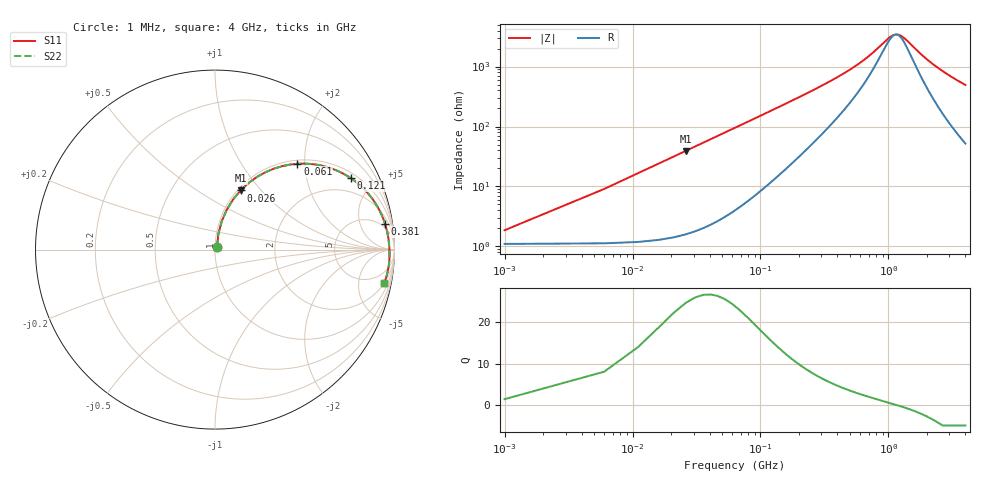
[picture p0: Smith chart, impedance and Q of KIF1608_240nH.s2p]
# MHz S RI R 50
!Freq ReS11 ImS11 ReS21 ImS21 ReS12 ImS12 ReS22 ImS22
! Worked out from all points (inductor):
!   801 points, 1 MHz to 4 GHz, reference 50 ohm
!   read as one part in series: L = 239 nH near 21 MHz
!   highest Q = 23.4 at 26 MHz (marker M1), where L = 239 nH
!   self-resonance near 1.146 GHz
!   S11 on the Smith chart (normalised r, x): 1 MHz: 1.02, +0.03; 26 MHz: 1.03, +0.78; 61 MHz: 1.08, +1.84; 121 MHz: 1.24, +3.66; 381 MHz: 4, +12; 4 GHz: 2, -10
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1  0.0111 0.0147  0.9889 -0.0147  0.9889 -0.0147  0.0111 0.0147
11  0.0374 0.1572  0.9626 -0.1572  0.9626 -0.1572  0.0374 0.1572
26  0.1424 0.3298  0.8576 -0.3298  0.8576 -0.3298  0.1424 0.3298
31  0.1877 0.3718  0.8123 -0.3718  0.8123 -0.3718  0.1877 0.3718
41  0.2829 0.4321  0.7171 -0.4321  0.7171 -0.4321  0.2829 0.4321
61  0.4594 0.4782  0.5406 -0.4782  0.5406 -0.4782  0.4594 0.4782
91  0.6467 0.4528  0.3533 -0.4528  0.3533 -0.4528  0.6467 0.4528
121  0.7572 0.3978  0.2428 -0.3978  0.2428 -0.3978  0.7572 0.3978
161  0.8386 0.3287  0.1614 -0.3287  0.1614 -0.3287  0.8386 0.3287
211  0.8907 0.2628  0.1093 -0.2628  0.1093 -0.2628  0.8907 0.2628
286  0.9273 0.1961  0.0727 -0.1961  0.0727 -0.1961  0.9273 0.1961
381  0.9476 0.1429  0.0524 -0.1429  0.0524 -0.1429  0.9476 0.1429
671  0.9661 0.0614  0.0339 -0.0614  0.0339 -0.0614  0.9661 0.0614
931  0.9703 0.0231  0.0297 -0.0231  0.0297 -0.0231  0.9703 0.0231
1066  0.9713 0.008  0.0287 -0.008  0.0287 -0.008  0.9713 0.008
1186  0.9718 -0.00388  0.0282 0.00388  0.0282 0.00388  0.9718 -0.00388
1336  0.9722 -0.0173  0.0278 0.0173  0.0278 0.0173  0.9722 -0.0173
1681  0.972 -0.0447  0.028 0.0447  0.028 0.0447  0.972 -0.0447
2001  0.9707 -0.0675  0.0293 0.0675  0.0293 0.0675  0.9707 -0.0675
2671  0.9647 -0.1109  0.0353 0.1109  0.0353 0.1109  0.9647 -0.1109
3336  0.9549 -0.15  0.0451 0.15  0.0451 0.15  0.9549 -0.15
4000  0.9424 -0.186  0.0576 0.186  0.0576 0.186  0.9424 -0.186
